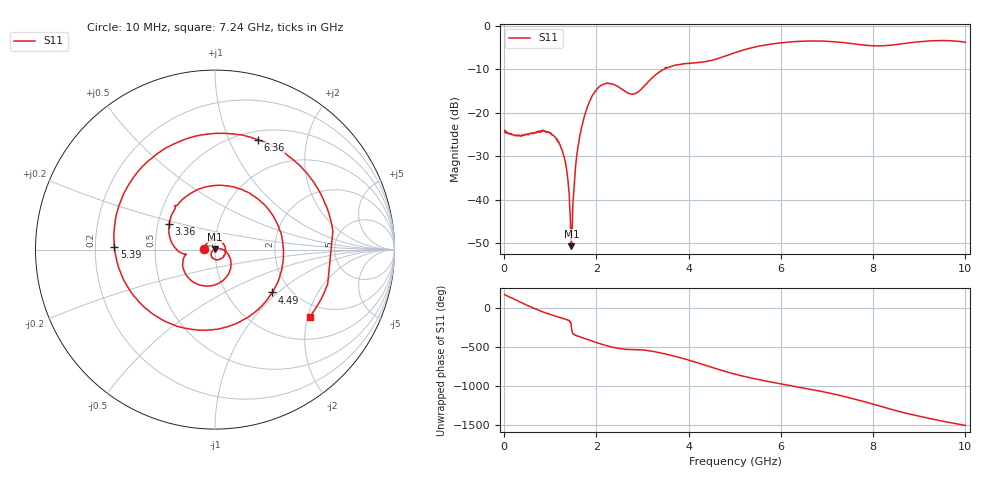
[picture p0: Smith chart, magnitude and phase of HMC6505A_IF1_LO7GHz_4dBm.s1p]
! Analog Devices, Inc.
! 1 Analog Way
! Wilmington, MA 01887
! http://www.analog.com
! Date:  2021-09-17 NN
! Board Name:  EV1HMC6505ALC5 (125487-1) with HMC6505ALC5 installed
! File Description:  S-Parameters for evaluation board without connectors or board loss de-embedded
! File Generation:  Calibrated Network Analyzer
! Chip Part Number:  HMC6505A
! Chip Description:  GaAs, MMIC, IQ Upconverter
! Chip Frequency:  5.5 to 8.6 GHz
! Chip Package:  LCC, 4.9 x 4.9 x 1 mm
! Chip State:
!  Temperature:  25C
!  LO Frequency:  7GHz
!  LO Power:  4dBm
! Note:
!  Analog Devices supplies this data as a sample of measured data at the evaluation board
!  ports for this product.  Your particular data for this product may vary.
!  Analog Devices reserves the right to change this data at anytime.
!  All lines below in this file are as is from the Network Analyzer.
!Keysight Technologies,N5245A,MY49151104,A.10.65.16
!Date: Tuesday, September 14, 2021 10:47:11
!Correction: S22(Full 2 Port(1,2))
!S1P File: Measurement: S22:
# Hz S  dB  R 50
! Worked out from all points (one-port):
!   980 points, 10 MHz to 10 GHz, reference 50 ohm
!   lowest |S11| = -50.6 dB at 1.46 GHz (marker M1), VSWR 1.01, Z = 49.9 + j0.283 ohm
!   |S11| at or under -10 dB: start of sweep to 3.473 GHz
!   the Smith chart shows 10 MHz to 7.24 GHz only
!   S11 on the Smith chart (normalised r, x): 10 MHz: 0.88, +0.00; 3.36 GHz: 0.57, +0.18; 4.49 GHz: 1.62, -0.92; 5.39 GHz: 0.28, +0.01; 6.36 GHz: 0.60, +1.28; 7.24 GHz: 1.60, -2.06
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1e7  -24.07 178.9
9.8e8  -24.58 -72.8
1.26e9  -28.64 -127.1
1.36e9  -33.47 -145.0
1.46e9  -50.65 104.8
1.6e9  -27.80 3.8
1.81e9  -18.49 -40.9
2.11e9  -13.65 -101.1
2.51e9  -14.27 -157.9
2.84e9  -15.59 -171.1
3.36e9  -10.68 151.0
3.76e9  -8.99 94.0
4.2e9  -8.49 18.2
4.49e9  -7.98 -36.8
5.01e9  -6.19 -127.8
5.39e9  -5.03 178.7
5.87e9  -4.12 121.8
6.26e9  -3.70 79.4
6.36e9  -3.66 68.7
6.84e9  -3.55 14.8
7.24e9  -3.78 -35.3
7.51e9  -4.10 -73.9
7.8e9  -4.47 -119.9
8.14e9  -4.65 -178.0
8.48e9  -4.37 125.1
8.76e9  -3.99 82.4
9.35e9  -3.45 5.7
1e10  -3.81 -68.2
